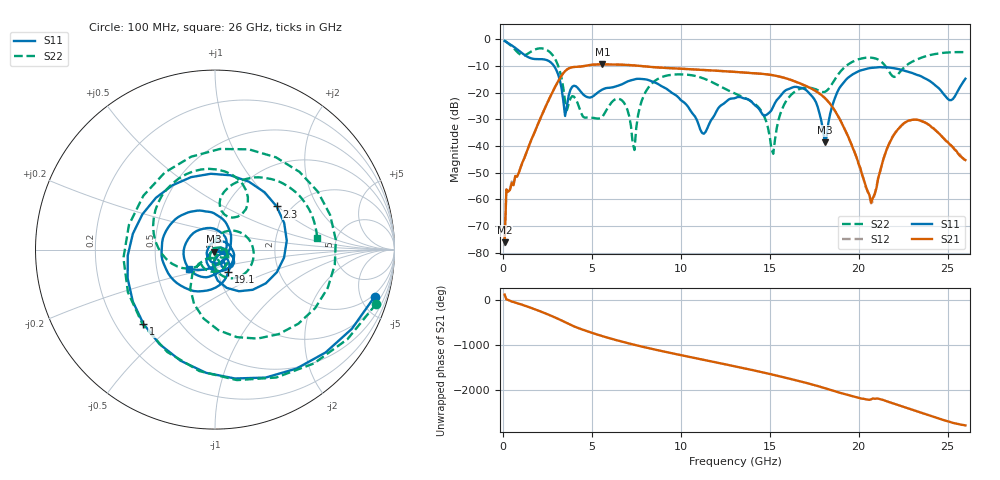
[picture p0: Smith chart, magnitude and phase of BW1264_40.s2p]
!Keysight Technologies,N5245B,MY57181159,A.13.60.06
!Date: Friday, December 18, 2020 23:54:09
!Correction: S11(Full 2 Port(1,2))
!S21(Full 2 Port(1,2))
!S12(Full 2 Port(1,2))
!S22(Full 2 Port(1,2))
!S2P File: Measurements: S11, S21, S12, S22:
# Hz S  dB  R 50
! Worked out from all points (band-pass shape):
!   260 points, 100 MHz to 26 GHz, reference 50 ohm
!   highest |S21| = -9.44 dB at 5.6 GHz (marker M1); lowest = -76.1 dB at 100 MHz (marker M2)
!   |S21| within 3 dB of the highest: 3.438 GHz to 13.47 GHz (10.03 GHz wide, 119 % of centre)
!   lowest |S11| = -38.7 dB at 18.1 GHz (marker M3), VSWR 1.02, Z = 49.5 - j1.05 ohm
!   |S11| at or under -10 dB: 2.872 GHz to end of sweep
!   |S22| runs from -43.0 to -0.5 dB; largest |S21 - S12| = 0.00053
!   S11 on the Smith chart (normalised r, x): 100 MHz: 1.73, -6.47; 1 GHz: 0.31, -0.39; 2.3 GHz: 1.69, +0.98; 19.1 GHz: 1.12, -0.29; 26 GHz: 0.73, -0.16
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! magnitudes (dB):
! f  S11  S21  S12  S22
! 100 MHz  -0.7  -76.1  -77.6  -0.5
! 200 MHz  -1.1  -56.3  -56.3  -1.0
! 1 GHz  -4.8  -48.1  -48.0  -5.8
! 2.3 GHz  -7.6  -26.8  -26.8  -3.6
! 3.5 GHz  -28.8  -12.0  -12.0  -23.3
! 4.5 GHz  -20.6  -10.1  -10.1  -29.0
! 5.6 GHz  -18.8  -9.4  -9.4  -29.0
! 6.7 GHz  -16.9  -9.6  -9.6  -23.0
! 7.4 GHz  -15.0  -9.8  -9.8  -41.5
! 7.8 GHz  -14.9  -10.1  -10.1  -23.2
! 8.8 GHz  -17.1  -10.6  -10.6  -14.6
! 11.3 GHz  -35.4  -11.5  -11.5  -14.7
! 13.1 GHz  -22.0  -12.3  -12.3  -20.5
! 15.2 GHz  -25.3  -13.5  -13.5  -43.0
! 15.9 GHz  -19.1  -14.6  -14.6  -23.5
! 17.4 GHz  -21.5  -18.7  -18.7  -18.4
! 18.1 GHz  -38.7  -22.0  -22.0  -19.7
! 19.1 GHz  -16.7  -32.1  -32.1  -11.2
! 20.7 GHz  -10.7  -61.3  -61.5  -6.9
! 21.7 GHz  -10.6  -39.3  -39.5  -12.0
! 23.4 GHz  -13.6  -30.4  -30.4  -7.2
! 26 GHz  -14.8  -45.3  -45.7  -4.8
